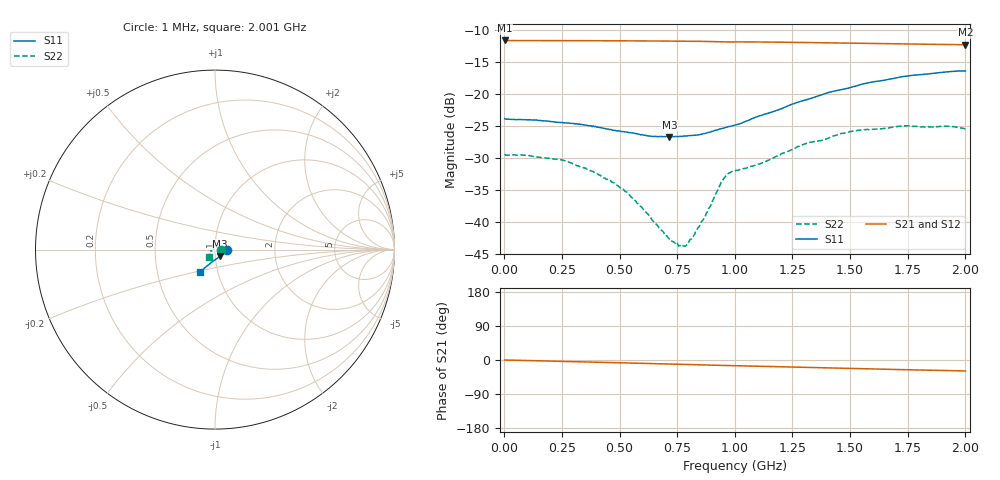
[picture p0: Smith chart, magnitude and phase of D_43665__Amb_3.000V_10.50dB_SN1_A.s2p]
! device id: 43665_
! dir: \\malibu\benchdata\1_engineers\tn_data\43665_75ohm\new\sparar\43665_\amb\3p000v\10p50db
! Serial: 1
! Insertion: A
! Temp: Amb
! VDD: 3.000V
! Attenuation Step: 10.50dB
! IDD: 1.449735e+00mA
! FILE NAME
! DATE 03-27-2009 08:35:56
! CORRECTED  DATA
#  Hz  S  RI  R  75
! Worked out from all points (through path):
!   401 points, 1 MHz to 2.001 GHz, reference 75 ohm
!   highest |S21| = -11.59 dB at 1 MHz (marker M1); lowest = -12.3 dB at 2.001 GHz (marker M2)
!   group delay of S21, straight-line fit = 40.8 ps
!   lowest |S11| = -26.7 dB at 716 MHz (marker M3), VSWR 1.10, Z = 79.2 - j5.81 ohm
!   |S11| at or under -10 dB: start of sweep to end of sweep
!   |S22| runs from -43.7 to -24.9 dB; largest |S21 - S12| = 0.00088
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1000000  0.0645 -0.000844  0.2633 -0.000544  0.2635 -0.0004  0.034 -0.000312
2.41e8  0.0594 -0.0104  0.262 -0.0159  0.2621 -0.016  0.0295 0.00909
3.36e8  0.0563 -0.0147  0.2613 -0.0223  0.2614 -0.0224  0.0243 0.0116
4.66e8  0.0484 -0.0208  0.2599 -0.0311  0.2601 -0.0311  0.0167 0.012
5.26e8  0.0444 -0.0248  0.2591 -0.0352  0.2592 -0.0352  0.013 0.0115
6.01e8  0.0385 -0.0289  0.2578 -0.04  0.2578 -0.0401  0.00675 0.0109
6.71e8  0.0323 -0.0337  0.2568 -0.0447  0.2567 -0.0447  0.00313 0.00851
7.16e8  0.0286 -0.0366  0.2559 -0.0478  0.256 -0.0478  0.000297 0.00739
7.56e8  0.0252 -0.0393  0.2551 -0.0507  0.2552 -0.0506  -0.00295 0.00581
7.91e8  0.0218 -0.0419  0.2543 -0.0531  0.2543 -0.0531  -0.00534 0.00395
8.16e8  0.0194 -0.0435  0.2537 -0.0548  0.2537 -0.0548  -0.00724 0.00199
8.71e8  0.0134 -0.0475  0.2521 -0.0588  0.252 -0.0586  -0.0106 -0.00269
9.51e8  0.00464 -0.054  0.2487 -0.0632  0.2488 -0.063  -0.0206 -0.00753
9.71e8  0.00271 -0.0557  0.2483 -0.064  0.2485 -0.0638  -0.023 -0.00674
1.001e9  -0.000794 -0.0573  0.248 -0.0654  0.2481 -0.0653  -0.0244 -0.0064
1.116e9  -0.0139 -0.067  0.2453 -0.073  0.2456 -0.0728  -0.0259 -0.013
1.336e9  -0.0376 -0.0857  0.2383 -0.0861  0.2387 -0.086  -0.032 -0.0277
1.511e9  -0.0554 -0.0997  0.2317 -0.0957  0.2321 -0.0959  -0.035 -0.0379
1.671e9  -0.0687 -0.1116  0.2258 -0.1037  0.2259 -0.1041  -0.0348 -0.0422
1.736e9  -0.0735 -0.1167  0.2232 -0.1067  0.2235 -0.1072  -0.0343 -0.0451
1.911e9  -0.0825 -0.1239  0.2168 -0.1141  0.2167 -0.1142  -0.0338 -0.0449
2.001e9  -0.0852 -0.1261  0.2135 -0.1177  0.2129 -0.1182  -0.0317 -0.0434
